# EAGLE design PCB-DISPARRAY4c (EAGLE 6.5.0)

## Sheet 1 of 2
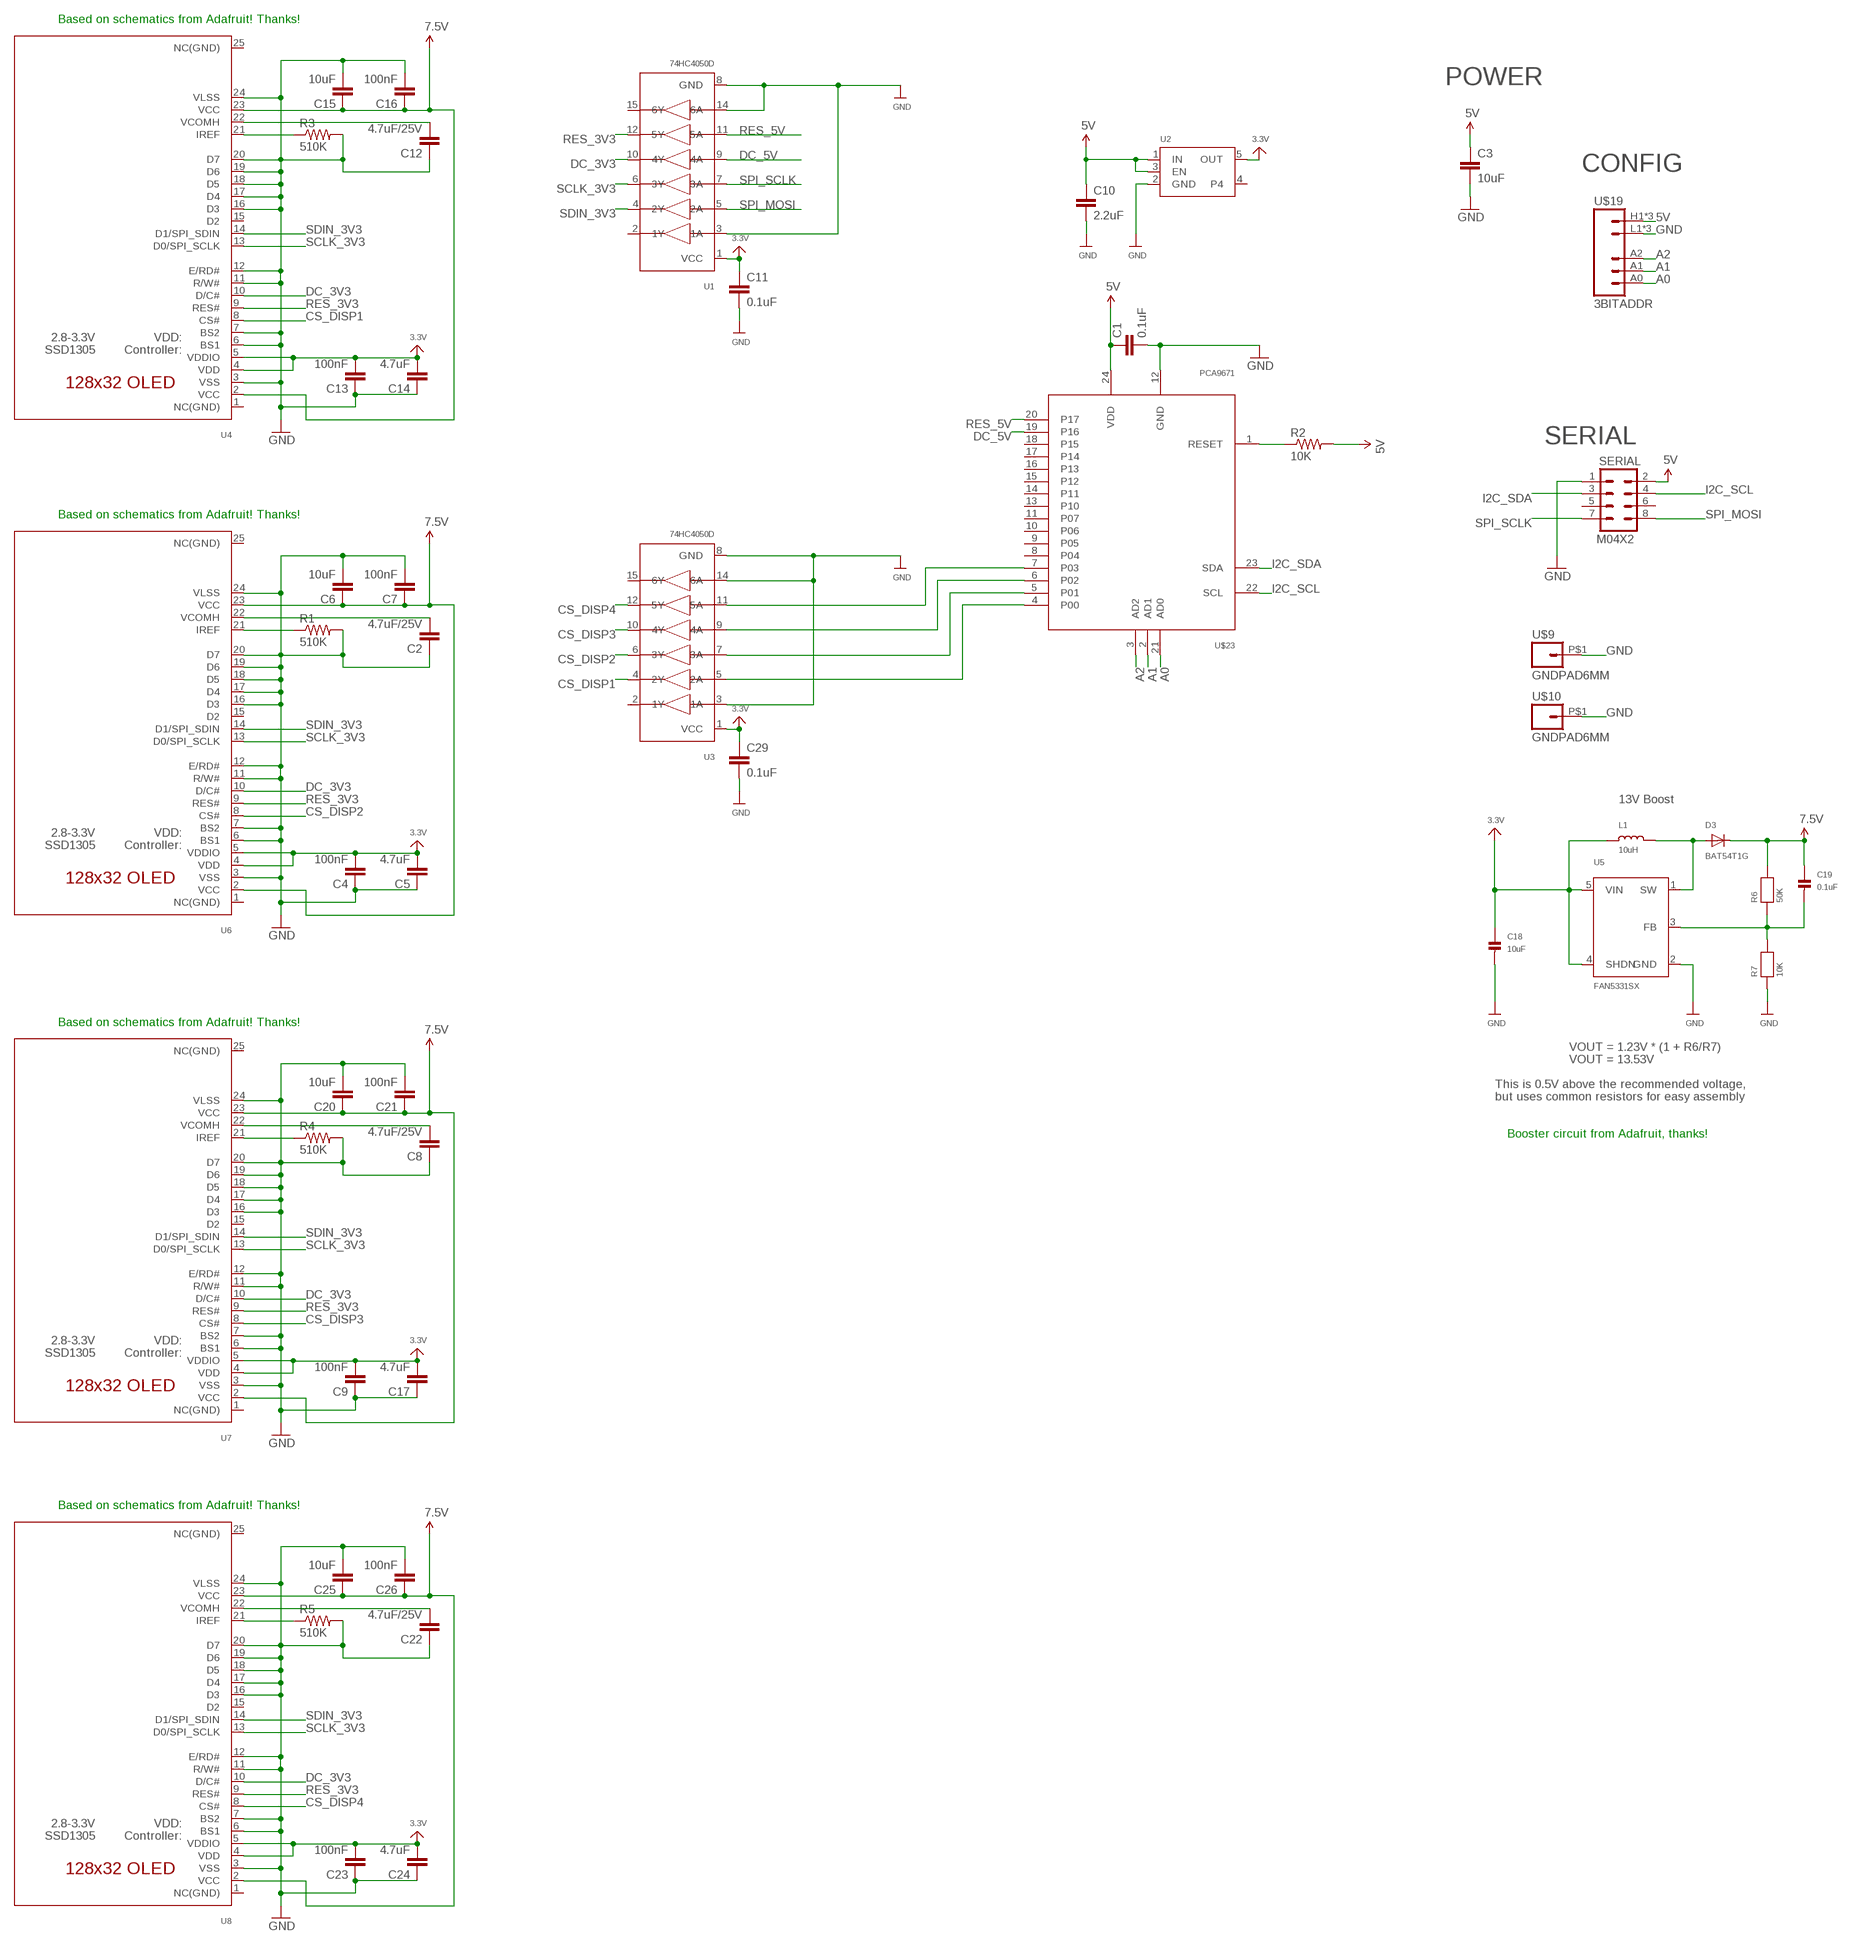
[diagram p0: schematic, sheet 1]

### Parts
C1  0.1uF  CAP0603-CAP  [0603-CAP]
C2  4.7uF/25V  CAP0805  [0805]
C3  10uF  CAP0805  [0805]
C4  100nF  CAP0603-CAP  [0603-CAP]
C5  4.7uF  CAP0603-CAP  [0603-CAP]
C6  10uF  CAP0603-CAP  [0603-CAP]
C7  100nF  CAP0603-CAP  [0603-CAP]
C8  4.7uF/25V  CAP0805  [0805]
C9  100nF  CAP0603-CAP  [0603-CAP]
C10  2.2uF  CAP0603-CAP  [0603-CAP]
C11  0.1uF  CAP0603-CAP  [0603-CAP]
C12  4.7uF/25V  CAP0805  [0805]
C13  100nF  CAP0603-CAP  [0603-CAP]
C14  4.7uF  CAP0603-CAP  [0603-CAP]
C15  10uF  CAP0603-CAP  [0603-CAP]
C16  100nF  CAP0603-CAP  [0603-CAP]
C17  4.7uF  CAP0603-CAP  [0603-CAP]
C18  10uF  CAP_CERAMIC0805  [0805]
C19  0.1uF  CAP_CERAMIC0805  [0805]
C20  10uF  CAP0603-CAP  [0603-CAP]
C21  100nF  CAP0603-CAP  [0603-CAP]
C22  4.7uF/25V  CAP0805  [0805]
C23  100nF  CAP0603-CAP  [0603-CAP]
C24  4.7uF  CAP0603-CAP  [0603-CAP]
C25  10uF  CAP0603-CAP  [0603-CAP]
C26  100nF  CAP0603-CAP  [0603-CAP]
C29  0.1uF  CAP0603-CAP  [0603-CAP]
D3  BAT54T1G  DIODESOD-123  [SOD-123]
L1  10uH  INDUCTOR  [INDUCTOR_1007]
R1  510K  RESISTOR0603-RES  [0603-RES]
R2  10K  RESISTOR0603-RES  [0603-RES]
R3  510K  RESISTOR0603-RES  [0603-RES]
R4  510K  RESISTOR0603-RES  [0603-RES]
R5  510K  RESISTOR0603-RES  [0603-RES]
R6  50K  RESISTOR0805  [0805]
R7  10K  RESISTOR0805  [0805]
SERIAL  M04X2  [2X4]
U1  74HC4050D  74HC4050DTSSOP16  [TSSOP16]
U2  VREG_SOT23-5  [SOT23-5]
U3  74HC4050D  74HC4050DTSSOP16  [TSSOP16]
U4  ER-OLED0.91-2  [ER-OLED0.91-2_WRAPAROUND]
U5  FAN5331SX  FAN5331  [SOT23-5]
U6  ER-OLED0.91-2  [ER-OLED0.91-2_WRAPAROUND]
U7  ER-OLED0.91-2  [ER-OLED0.91-2_WRAPAROUND]
U8  ER-OLED0.91-2  [ER-OLED0.91-2_WRAPAROUND]
U$9  GNDPAD6MM  [3.2MMPAD6MM]
U$10  GNDPAD6MM  [3.2MMPAD6MM]
U$19  3BITADDR  [3BITADDR]
U$23  PCA9671  [TSSOP24]

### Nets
3.3V: C4.2 C5.2 C9.2 C11.1 C13.2 C14.2 C17.2 C18.1 C23.2 C24.2 C29.1 L1.P$1 U1.1(VCC) U2.5(OUT) U3.1(VCC) U4.4(VDD) U4.5(VDDIO) U5.4(SHDN) U5.5(VIN) U6.4(VDD) U6.5(VDDIO) U7.4(VDD) U7.5(VDDIO) U8.4(VDD) U8.5(VDDIO)
5V [Power]: C1.1 C3.1 C10.1 R2.2 SERIAL.2 U2.1(IN) U2.3(EN) U$19.H1(VCC) U$19.H2(VCC) U$19.H3(VCC) U$23.24(VDD)
7.5V [Power]: C6.1 C7.1 C15.1 C16.1 C19.1 C20.1 C21.1 C25.1 C26.1 D3.C R6.2 U4.2(VCC) U4.23(VCC) U6.2(VCC) U6.23(VCC) U7.2(VCC) U7.23(VCC) U8.2(VCC) U8.23(VCC)
A0: U$19.A0 U$23.21(AD0)
A1: U$19.A1 U$23.2(AD1)
A2: U$19.A2 U$23.3(AD2)
CS_DISP1: U3.4(2Y) U4.8(CS#)
CS_DISP2: U3.6(3Y) U6.8(CS#)
CS_DISP3: U3.10(4Y) U7.8(CS#)
CS_DISP4: U3.12(5Y) U8.8(CS#)
DC_3V3: U1.10(4Y) U4.10(D/C#) U6.10(D/C#) U7.10(D/C#) U8.10(D/C#)
DC_5V: U1.9(4A) U$23.19(P16)
GND [Power]: C1.2 C2.1 C3.2 C4.1 C5.1 C6.2 C7.2 C8.1 C9.1 C10.2 C11.2 C12.1 C13.1 C14.1 C15.2 C16.2 C17.1 C18.2 C20.2 C21.2 C22.1 C23.1 C24.1 C25.2 C26.2 C29.2 R1.2 R3.2 R4.2 R5.2 R7.1 SERIAL.1 U1.3(1A) U1.8(GND) U1.14(6A) U2.2(GND) U3.3(1A) U3.8(GND) U3.14(6A) U4.3(VSS) U4.6(BS1) U4.7(BS2) U4.11(R/W#) U4.12(E/RD#) U4.16(D3) U4.17(D4) U4.18(D5) U4.19(D6) U4.20(D7) U4.24(VLSS) U5.2(GND) U6.3(VSS) U6.6(BS1) U6.7(BS2) U6.11(R/W#) U6.12(E/RD#) U6.16(D3) U6.17(D4) U6.18(D5) U6.19(D6) U6.20(D7) U6.24(VLSS) U7.3(VSS) U7.6(BS1) U7.7(BS2) U7.11(R/W#) U7.12(E/RD#) U7.16(D3) U7.17(D4) U7.18(D5) U7.19(D6) U7.20(D7) U7.24(VLSS) U8.3(VSS) U8.6(BS1) U8.7(BS2) U8.11(R/W#) U8.12(E/RD#) U8.16(D3) U8.17(D4) U8.18(D5) U8.19(D6) U8.20(D7) U8.24(VLSS) U$9.P$1 U$10.P$1 U$19.L1(GND) U$19.L2(GND) U$19.L3(GND) U$23.12(GND)
I2C_SCL: SERIAL.4 U$23.22(SCL)
I2C_SDA: SERIAL.3 U$23.23(SDA)
N$1: R2.1 U$23.1(RESET)
N$2: R1.1 U6.21(IREF)
N$3: C2.2 U6.22(VCOMH)
N$4: R4.1 U7.21(IREF)
N$5: R3.1 U4.21(IREF)
N$6: C8.2 U7.22(VCOMH)
N$7: R5.1 U8.21(IREF)
N$8: C22.2 U8.22(VCOMH)
N$10: C12.2 U4.22(VCOMH)
N$14: D3.A L1.P$2 U5.1(SW)
N$15: C19.2 R6.1 R7.2 U5.3(FB)
N$29: U3.5(2A) U$23.4(P00)
N$30: U3.7(3A) U$23.5(P01)
N$31: U3.9(4A) U$23.6(P02)
N$32: U3.11(5A) U$23.7(P03)
RES_3V3: U1.12(5Y) U4.9(RES#) U6.9(RES#) U7.9(RES#) U8.9(RES#)
RES_5V: U1.11(5A) U$23.20(P17)
SCLK_3V3: U1.6(3Y) U4.13(D0/SPI_SCLK) U6.13(D0/SPI_SCLK) U7.13(D0/SPI_SCLK) U8.13(D0/SPI_SCLK)
SDIN_3V3: U1.4(2Y) U4.14(D1/SPI_SDIN) U6.14(D1/SPI_SDIN) U7.14(D1/SPI_SDIN) U8.14(D1/SPI_SDIN)
SPI_MOSI: SERIAL.8 U1.5(2A)
SPI_SCLK: SERIAL.7 U1.7(3A)
Unconnected: SERIAL.5 SERIAL.6 U1.2(1Y) U1.15(6Y) U2.4 U3.2(1Y) U3.15(6Y) U4.1(NC(GND)) U4.15(D2) U4.25(NC(GND)) U6.1(NC(GND)) U6.15(D2) U6.25(NC(GND)) U7.1(NC(GND)) U7.15(D2) U7.25(NC(GND)) U8.1(NC(GND)) U8.15(D2) U8.25(NC(GND)) U$23.8(P04) U$23.9(P05) U$23.10(P06) U$23.11(P07) U$23.13(P10) U$23.14(P11) U$23.15(P12) U$23.16(P13) U$23.17(P14) U$23.18(P15)

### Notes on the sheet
- Based on schematics from Adafruit! Thanks!
- POWER
- CONFIG
- SERIAL
- Based on schematics from Adafruit! Thanks!
- 13V Boost
- Based on schematics from Adafruit! Thanks!
- VOUT = 1.23V * (1 + R6/R7)
- VOUT = 13.53V
- This is 0.5V above the recommended voltage,
- but uses common resistors for easy assembly
- Booster circuit from Adafruit, thanks!
- Based on schematics from Adafruit! Thanks!

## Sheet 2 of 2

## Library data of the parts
C1-C17 C20-C26 C29 = SparkFun:CAP: Capacitor
C18 C19 = microbuilder:CAP_CERAMIC: Ceramic Capacitors
D3 = microbuilder:DIODE: Diode
L1 = microbuilder:INDUCTOR: Inductors
R1-R5 = SparkFun:RESISTOR: Resistor
R6 R7 = microbuilder:RESISTOR: Resistors
SERIAL = SparkFun:M04X2
U1 U3 = SKAARHOJ:74HC4050D: 6-channel level shifter 74HC4050D - 2V-6V Supply Digikey: 74HC4050D,653-ND Mouser: 771-74HC4050D-T
U2 = microbuilder:VREG_SOT23-5: SOT23-5 Fixed Voltage Regulators To better organise some of the SOT23-5 fixed voltage regulators in this library, this new part was created. Part Current Out V Out V In V Dropout Digikey Part No. ADP121 150mA 3.3V 3.4-5.5V 0.09V @ 150mA ADP121-AUJZ33R7CT-ND ADP121 150mA 3.0V 3.1-5.5V 0.09V @ 150mA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
U4 U6-U8 = SKAARHOJ:ER-OLED0.91-2: UG-2864HSWEG01 OLED display Both 1.3" and 0.96" models share the same FPC tab footprint, only the screen dimensions vary.
U5 = microbuilder:FAN5331: FAN5331 - LED/OLED 20V Boost Converter Digikey: FAN5331SXCT-ND
U$9 U$10 = SKAARHOJ:GNDPAD
U$19 = SKAARHOJ:3BITADDR
U$23 = SKAARHOJ:PCA9671

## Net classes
0 default: width 0.203 mm, drill 0.305 mm, clearance 0.152 mm
1 Power: width 0.203 mm, drill 0.406 mm, clearance 0.152 mm

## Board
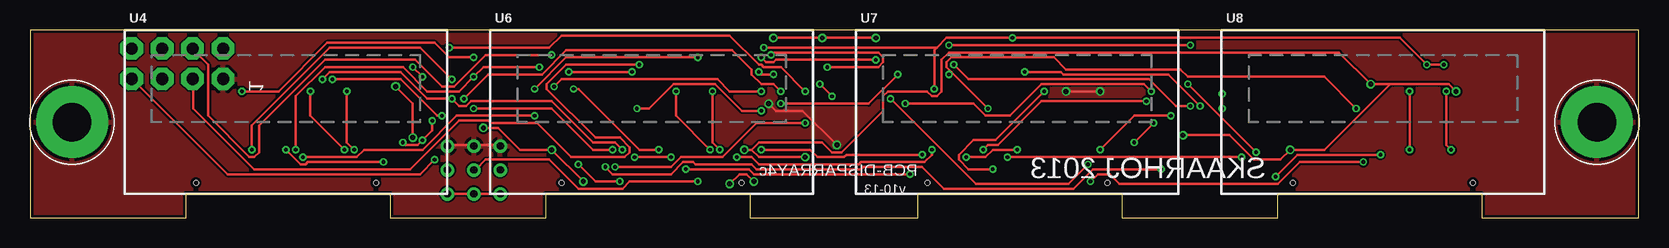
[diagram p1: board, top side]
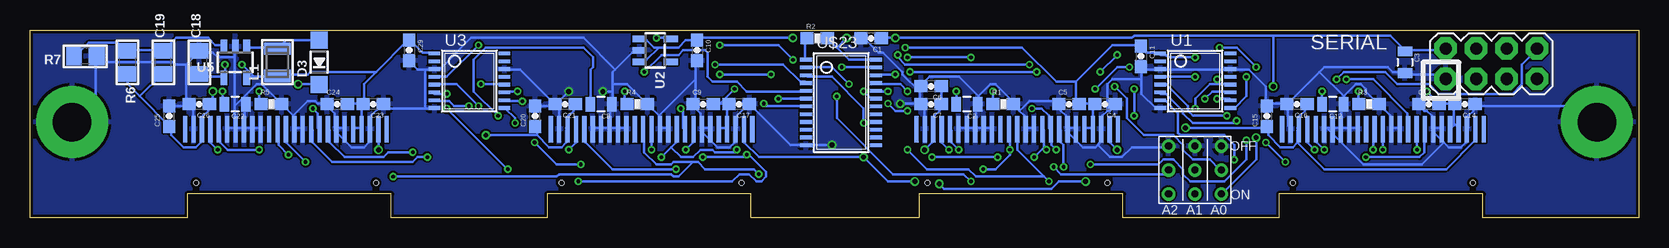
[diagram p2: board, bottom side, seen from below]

Size 134.11 x 15.7 mm. Coordinates in mm from the lower left corner, seen from the top.
Outline: 134.11,0 134.11,15.7 0,15.7 0,0 13,0 13,2 30,2 30,0 43,0 43,2 60,2 60,0 74,0 74,2 91,2 91,0 104,0 104,2 121,2 121,0 134.11,0
Copper layers (1*16): Top 0.035mm / dielectric 1.5mm / Bottom 0.035mm
Design rules "Fusion_eagle_rule_v1.1": minimum track width 6mil, minimum drill 12mil, track to track 6mil, track to pad 6mil, pad to pad 6mil, via to via 6mil, smd to smd 0mil, copper to edge 10mil, drill to drill 10mil, minimum pad ring 10mil, minimum via ring 6mil, stop-mask expansion 2mil, vias tented up to drill 100mil, thermal gap 10mil

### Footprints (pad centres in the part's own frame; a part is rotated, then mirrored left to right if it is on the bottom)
0603-CAP = smd 1.1 x 1: 1 -0.85,0; 2 0.85,0
0805 = smd 0.8 x 1.2: 1 -0.9,0; 2 0.9,0
0805' = smd 1.3 x 1.5: 1 -0.95,0; 2 0.95,0
SOD-123 = smd 1.4 x 1.4: A 1.85,0; C -1.85,0
INDUCTOR_1007 = smd 1.016 x 2.2: P$1 -1.127,0; P$2 1.127,0
0603-RES = smd 1.1 x 1: 1 -0.85,0; 2 0.85,0
2X4 = drill 1.016 pad 1.88 octagon: 1 -3.81,-1.27; 2 -3.81,1.27; 3 -1.27,-1.27; 4 -1.27,1.27; 5 1.27,-1.27; 6 1.27,1.27; 7 3.81,-1.27; 8 3.81,1.27
TSSOP16 = smd 0.305 x 0.991: 1 -3.575,-2.918; 2 -2.925,-2.918; 3 -2.275,-2.918; 4 -1.625,-2.918; 5 -0.975,-2.918; 6 -0.325,-2.918; 7 0.325,-2.918; 8 0.975,-2.918; 9 0.975,2.918; 10 0.325,2.918; 11 -0.325,2.918; 12 -0.975,2.918; 13 -1.625,2.918; 14 -2.275,2.918; 15 -2.925,2.918; 16 -3.575,2.918
SOT23-5 = smd 0.55 x 1.2: 1 -0.95,-1.3; 2 0,-1.3; 3 0.95,-1.3; 4 0.95,1.3; 5 -0.95,1.3
ER-OLED0.91-2_WRAPAROUND = smd 0.35 x 2.2 bottom: 1 -8.4,-1.43; 2 -7.7,-1.43; 3 -7,-1.43; 4 -6.3,-1.43; 5 -5.6,-1.43; 6 -4.9,-1.43; 7 -4.2,-1.43; 8 -3.5,-1.43; 9 -2.8,-1.43; 10 -2.1,-1.43; 11 -1.4,-1.43; 12 -0.7,-1.43; 13 0,-1.43; 14 0.7,-1.43; 15 1.4,-1.43; 16 2.1,-1.43; 17 2.8,-1.43; 18 3.5,-1.43; 19 4.2,-1.43; 20 4.9,-1.43; 21 5.6,-1.43; 22 6.3,-1.43; 23 7,-1.43; 24 7.7,-1.43; 25 8.4,-1.43 | hole 0.4: -7.5,-5.93; 7.5,-5.93
3.2MMPAD6MM = drill 3.2 pad 6: P$1 0,0
3BITADDR = drill 0.6: A0 -2.2,0; A1 0,0; A2 2.2,0; H1 -2.2,2; H2 0,2; H3 2.2,2; L1 -2.2,-2; L2 0,-2; L3 2.2,-2
TSSOP24 = smd 0.305 x 0.991: 1 -4.225,-2.918; 2 -3.575,-2.918; 3 -2.925,-2.918; 4 -2.275,-2.918; 5 -1.625,-2.918; 6 -0.975,-2.918; 7 -0.325,-2.918; 8 0.325,-2.918; 9 0.975,-2.918; 10 1.625,-2.918; 11 2.275,-2.918; 12 2.925,-2.918; 13 2.925,2.918; 14 2.275,2.918; 15 1.625,2.918; 16 0.975,2.918; 17 0.325,2.918; 18 -0.325,2.918; 19 -0.975,2.918; 20 -1.625,2.918; 21 -2.275,2.918; 22 -2.925,2.918; 23 -3.575,2.918; 24 -4.225,2.918

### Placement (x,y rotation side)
C1  64,15 180 bottom
C2  56,9.5 180 bottom
C3  19.5,13 270 bottom
C4  44.5,9.5 180 bottom
C5  47.5,9.5 0 bottom
C6  59,11 180 bottom
C7  59,9.5 180 bottom
C8  86.5,9.5 180 bottom
C9  78,9.5 0 bottom
C10  78.5,14 270 bottom
C11  41.5,13.5 270 bottom
C12  25.5,9.5 180 bottom
C13  17.5,9.5 0 bottom
C14  14.5,9.5 180 bottom
C15  31,8.5 90 bottom
C16  28.5,9.5 180 bottom
C17  75,9.5 180 bottom
C18  10uF  [0805']  120,13 90 bottom
C19  0.1uF  [0805']  123,13 90 bottom
C20  92,8.5 90 bottom
C21  89.5,9.5 180 bottom
C22  117,9.5 180 bottom
C23  105.5,9.5 180 bottom
C24  108.5,9.5 0 bottom
C25  122.5,8.5 90 bottom
C26  120,9.5 180 bottom
C29  102.5,14 270 bottom
D3  110,13 90 bottom
L1  113.5,13 90 bottom
R1  53,9.5 0 bottom
R2  68.5,15 0 bottom
R3  22.5,9.5 0 bottom
R4  83.5,9.5 0 bottom
R5  114,9.5 0 bottom
R6  50K  [0805']  126,13 270 bottom
R7  10K  [0805']  129.5,13.5 180 bottom
SERIAL  12.29,12.88 0 bottom
U1  36.98,10.16 270 bottom
U2  82,14 270 bottom
U3  97.49,10.16 270 bottom
U4  21.34,8.85 0 top
U5  117,13 180 bottom
U6  51.82,8.85 0 top
U7  82.3,8.85 0 top
U8  112.78,8.85 0 top
U$9  130.61,8 0 top
U$10  3.5,8 0 top
U$19  37,4 180 bottom
U$23  66.5,8.99 270 bottom

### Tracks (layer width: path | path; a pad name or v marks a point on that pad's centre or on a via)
3.3V  (via drill 0.3)
  Top 0.203: v17.68,10.57 20.73,10.57 24.79,14.63 33.73,14.63 34.95,13.41 v36.98,13.41 | 75.59,14.22 75.39,14.02 v75.39,10.77 | 75.59,14.22 76.4,15.04 v81.89,15.04 114.2,15.04 v116.43,12.8 v117.86,12.8 | 75.59,14.22 v61.16,14.22
  Bottom 0.203: 15.44,7.92 15.44,7.72 15.65,7.52 U4.5 | 15.44,7.92 15.44,9.35 C14.2 15.44,9.55 16.46,9.55 C13.2 16.66,9.55 v17.68,10.57 | 15.44,7.92 15.04,7.52 U4.4 | 45.52,7.52 45.52,9.35 C4.2 45.52,9.55 46.53,9.55 C5.2 46.74,9.55 46.94,9.75 46.94,11.38 | 46.94,11.38 43.89,14.43 41.66,14.43 C11.1 41.45,14.22 41.05,13.82 40.03,13.82 U1.1 39.83,13.61 39.42,13.61 39.22,13.41 v36.98,13.41 | 45.52,7.52 46.13,7.52 U6.5 | 45.52,7.52 U6.4 | 76,7.52 76.61,7.52 U7.5 | 76.61,9.55 77.01,9.55 C9.2 76.61,9.55 | 76.61,9.55 76,9.55 C17.2 76,9.35 76,7.52 | v81.89,15.04 80.87,15.04 U2.5 | 76.61,9.55 v75.39,10.77 | 76,7.52 U7.4 | C18.1 119.89,11.99 119.69,11.79 118.06,11.79 U5.4 117.86,11.79 v117.86,12.8 | 115.42,11.79 113.59,11.79 L1.P$1 113.39,11.99 110.95,11.99 110.74,12.19 105.26,12.19 | 115.42,11.79 116.03,11.79 U5.5 | 115.42,11.79 v116.43,12.8 | U3.1 100.58,13.82 101.4,13.82 102.41,14.83 C29.1 102.62,14.83 105.26,12.19 | C23.2 106.48,9.55 107.49,9.55 C24.2 | 106.48,7.52 106.48,9.35 C23.2 | 105.26,12.19 106.27,11.18 106.27,9.55 C23.2 | 106.48,7.52 107.09,7.52 U8.5 | 106.48,7.52 U8.4 | 46.94,11.38 48.56,11.38 51.41,14.22 v61.16,14.22
5V  (via drill 0.41)
  Top 0.203: U$19.H1 34.95,2.03 36.98,2.03 U$19.H2 37.19,2.03 39.01,2.03 U$19.H3 | v61.98,15.04 v66.04,15.04 v70.51,15.04 | v31.9,6.71 31.9,9.55 v30.48,10.97
  Bottom 0.203: 81.69,14.22 82.09,14.22 82.7,14.83 83.11,14.83 U2.1 | 81.69,14.22 80.06,14.22 79.45,14.83 78.64,14.83 C10.1 78.44,15.04 v70.51,15.04 | 81.69,14.22 82.7,13.21 83.11,13.21 U2.3 | 66.85,14.22 67.46,14.83 R2.2 | 66.85,14.22 65.84,13.21 63.6,13.21 U$23.24 | 30.48,15.24 20.73,15.24 19.51,14.02 C3.1 19.3,14.02 16.26,14.02 SERIAL.2 | 30.48,15.24 42.06,15.24 42.27,15.04 v61.98,15.04 62.99,15.04 C1.1 | v66.04,15.04 66.85,14.22 | v31.9,6.71 31.9,4.88 34.75,2.03 U$19.H1 | 30.48,15.24 v30.48,10.97
7.5V  (via drill 0.41)
  Top 0.203: v37.8,7.52 39.01,7.52 40.84,5.69 v43.48,5.69 v46.13,3.05 | v64.62,5.08 60.76,5.08 60.15,5.69 | v59.54,5.69 60.15,5.69 | 113.39,11.18 118.26,11.18 v118.87,10.57 | 113.39,11.18 v111.76,11.18 109.12,13.82 76.61,13.82 76,13.21 76,10.57 75.59,10.16 75.18,10.16 74.78,10.57 71.53,10.57 71.12,10.16 71.12,8.94 67.67,5.49 66.85,5.49 66.04,6.3 60.76,6.3 60.15,5.69 | 113.39,11.18 107.9,5.69 v105.05,5.69 104.24,4.88 102.01,4.88 99.97,6.91 v96.11,6.91 | v58.32,2.85 59.13,3.66 59.74,3.66 v60.35,3.05
  Bottom 0.203: 44.09,7.52 U6.2 44.09,7.32 44.09,6.3 v43.48,5.69 | 28.45,6.3 28.85,5.89 29.87,5.89 30.89,6.91 30.89,7.52 C15.1 31.09,7.52 v37.8,7.52 | 28.45,6.3 28.45,7.32 U4.23 | C16.1 27.84,9.35 27.84,8.94 28.25,8.53 28.25,7.52 U4.23 | 28.45,6.3 26.21,4.06 16.05,4.06 13.61,6.5 13.61,7.32 U4.2 | 28.45,7.52 U4.23 | 74.57,7.52 U7.2 74.57,7.32 74.57,6.3 73.36,5.08 v64.62,5.08 62.59,3.05 v60.35,3.05 | C6.1 58.12,10.97 58.12,9.55 C7.1 58.32,9.35 58.32,8.94 58.73,8.53 58.73,7.52 U6.23 | 58.93,7.52 U6.23 | v59.54,5.69 58.93,6.3 58.93,7.32 U6.23 | 124.97,10.16 125.98,11.18 125.98,11.99 R6.2 | 124.97,10.16 122.53,7.72 C25.1 122.33,7.52 122.33,6.91 121.31,5.89 120.29,5.89 119.89,6.3 119.89,7.32 U8.23 | 124.97,10.16 123.14,11.99 C19.1 | 91.85,6.91 91.85,7.52 C20.1 | 91.85,6.91 90.83,5.89 89.81,5.89 89.41,6.3 89.41,7.32 U7.23 | C21.1 88.8,9.35 88.8,8.94 89.2,8.53 89.2,7.52 U7.23 | 89.41,7.52 U7.23 | 105.05,7.52 U8.2 105.05,7.32 v105.05,5.69 | U8.23 119.69,7.52 119.69,8.53 119.28,8.94 119.28,9.35 C26.1 119.08,9.55 118.87,9.75 v118.87,10.57 | v111.76,11.18 110.13,11.18 D3.C | 119.89,7.52 U8.23 | v96.11,6.91 91.85,6.91 | v46.13,3.05 48.36,3.05 48.97,2.44 57.91,2.44 v58.32,2.85
A0  (via drill 0.3)
  Top 0.203: v60.96,10.57 58.32,10.57 57.3,11.58 44.3,11.58 v43.69,10.97
  Bottom 0.203: v60.96,10.57 61.57,11.18 63.4,11.18 U$23.21 | v43.69,10.97 42.67,9.96 42.67,8.33 41.25,6.91 38.81,6.91 38,6.1 38,5.69 37.19,4.88 35.76,4.88 34.95,4.06 U$19.A0
A1  (via drill 0.3)
  Top 0.203: v66.85,10.16 v65.84,11.18 | v55.68,3.05 49.99,3.05 49.38,2.44 45.72,2.44 43.28,4.88 38,4.88 37.19,4.06 U$19.A1
  Bottom 0.203: v65.84,11.18 67.26,12.6 69.29,12.6 U$23.2 | v66.85,10.16 66.85,8.33 62.18,3.66 56.29,3.66 v55.68,3.05
A2  (via drill 0.3)
  Top 0.203: v64.62,7.92 60.55,7.92 57.71,5.08 54.25,5.08 53.44,4.27 v48.77,4.27
  Bottom 0.203: v64.62,7.92 64.62,9.14 67.26,11.79 69.29,11.79 U$23.3 | v48.77,4.27 48.16,3.66 39.42,3.66 39.22,3.86 U$19.A2
CS_DISP1  (via drill 0.3)
  Top 0.203: v76.61,14.43 v96.72,14.43 | v70.51,13.21 62.18,13.21 61.98,13.01 61.37,13.01 v60.96,13.41 | v55.68,13.41 44.7,13.41 v42.06,10.77 | v42.06,8.53 35.56,8.53 32.72,5.69 27.84,5.69 27.23,5.08 v22.76,5.08
  Bottom 0.203: v96.72,14.43 99.36,11.79 100.38,11.79 U3.4 | v76.61,14.43 71.73,14.43 v70.51,13.21 | v55.68,13.41 v60.96,13.41 | v42.06,8.53 v42.06,10.77 | v22.76,5.08 18.29,5.08 17.88,5.49 17.88,7.32 U4.8
CS_DISP2  (via drill 0.3)
  Top 0.203: v99.36,9.14 v99.36,10.36 | v94.28,4.06 88.59,4.06 86.97,2.44 76.2,2.44 74.37,4.27 69.49,4.27 69.29,4.06 60.55,4.06 60.15,4.47 55.47,4.47 55.27,4.67 54.46,4.67 53.44,3.66 48.56,3.66 v47.95,4.27
  Bottom 0.203: v99.36,10.36 100.38,10.36 U3.6 | v94.28,4.06 v99.36,9.14 | v47.95,4.27 47.95,6.1 48.16,6.3 48.16,7.32 U6.8
CS_DISP3  (via drill 0.3)
  Top 0.203: v93.07,9.75 84.33,9.75 80.67,6.1 79.86,6.1 v79.45,5.69
  Bottom 0.203: v93.07,9.75 94.49,9.75 U3.10 | v79.45,5.69 78.84,6.3 78.84,7.32 U7.8
CS_DISP4  (via drill 0.3)
  Top 0.203: v102.21,5.49 v96.52,11.18
  Bottom 0.203: v96.52,11.18 94.69,11.18 U3.12 | v102.21,5.49 104.24,5.49 104.65,5.08 107.9,5.08 109.12,6.3 109.12,7.32 U8.8
DC_3V3  (via drill 0.3)
  Top 0.203: v100.99,5.08 v81.48,5.08 | v24.38,11.58 24.99,12.19 30.89,12.19 33.12,9.96 v35.15,9.96 35.76,9.35 36.37,9.35 36.78,9.75 43.48,9.75 46.94,6.3 48.77,6.3 v49.38,5.69 | v75.18,5.69 75.18,5.28 74.57,4.67 69.29,4.67 69.09,4.47 60.76,4.47 60.15,5.08 v58.93,5.08 | v50.39,5.08 v53.44,5.08
  Bottom 0.203: v81.48,5.08 80.67,5.89 | 80.67,5.89 80.26,6.3 80.26,7.32 U7.10 | v100.99,5.08 101.8,5.08 102.21,4.67 108.92,4.67 110.54,6.3 110.54,7.32 U8.10 | v35.15,9.96 34.14,9.96 U1.10 | v24.38,11.58 22.15,11.58 19.3,8.74 19.3,7.52 U4.10 | 49.58,5.89 49.58,7.32 U6.10 | 80.67,5.89 79.86,5.08 78.84,5.08 78.23,5.69 77.22,5.69 77.01,5.49 75.39,5.49 v75.18,5.69 | v53.44,5.08 v58.93,5.08 | 49.58,5.89 v50.39,5.08 | 49.58,5.89 v49.38,5.69
DC_5V  (via drill 0.3)
  Top 0.203: v31.9,12.6 v32.72,11.79 | v34.95,14.22 43.28,14.22 44.3,15.24 58.32,15.24 60.76,12.8 60.96,12.8 61.16,12.6 62.59,12.6 v64.62,10.57
  Bottom 0.203: v32.72,11.79 32.72,10.16 33.73,9.14 33.93,9.14 U1.9 | v31.9,12.6 33.53,14.22 v34.95,14.22 | v64.62,10.57 64.01,9.96 63.6,9.96 U$23.19
GND  (via drill 0.41)
  Top 0.203: v86.36,10.57 v89.2,10.57 | U$19.L1 34.95,6.1 36.98,6.1 U$19.L2 37.19,6.1 39.01,6.1 U$19.L3 | v67.26,6.1 64.41,8.94 62.18,8.94 v61.57,9.55
  Bottom 0.203: U3.14 94.49,12.39 93.27,12.39 90.42,9.55 C21.2 | C20.2 91.85,9.35 90.42,9.35 C21.2 | U7.24 90.02,7.52 90.02,9.14 90.22,9.35 C21.2 | U7.16 84.53,7.52 84.94,7.52 U7.17 85.14,7.52 85.75,7.52 | 85.75,7.52 85.75,9.35 C8.1 85.55,9.55 85.55,10.57 | 85.34,12.39 85.55,12.19 85.55,11.18 | 85.34,12.39 83.92,13.82 83.31,13.82 U2.2 | 85.55,10.57 85.55,11.18 | U7.20 87.17,7.52 86.56,7.52 U7.19 86.36,7.52 85.95,7.52 U7.18 85.75,7.52 | v89.2,10.57 90.22,9.55 C21.2 | 85.55,10.57 v86.36,10.57 | 81.69,8.53 82.5,9.35 R4.2 82.7,9.55 84.33,11.18 85.55,11.18 | 81.69,8.53 81.69,7.52 U7.12 81.48,7.52 80.87,7.52 U7.11 | 78.64,9.14 78.23,8.74 78.23,7.52 U7.7 | 78.64,9.14 78.84,9.35 C9.1 78.64,9.14 | 78.64,9.14 78.64,11.58 | 78.64,11.58 78.64,13.01 C10.2 | U7.6 77.42,7.52 78.03,7.52 U7.7 | 78.64,11.58 81.69,8.53 | U7.7 78.23,7.32 76.81,5.89 75.79,5.89 75.39,6.3 75.39,7.32 U7.3 75.18,7.52 75.18,8.53 74.17,9.55 C17.1 73.97,9.35 70.71,6.1 69.49,6.1 U$23.12 69.29,6.1 v67.26,6.1 | 101.19,12.39 101.8,12.39 102.41,13.01 C29.2 | 101.19,12.39 100.58,12.39 U3.3 100.38,12.39 99.97,12.39 97.33,15.04 87.99,15.04 85.34,12.39 | 101.19,9.14 104.44,9.14 104.65,9.35 C23.1 104.85,9.35 105.66,8.53 105.66,7.52 U8.3 105.87,7.32 105.87,6.3 106.27,5.89 107.29,5.89 108.71,7.32 U8.7 | 101.19,9.14 100.58,9.14 U3.8 | 101.19,9.14 101.19,12.39 | 121.11,9.35 120.9,9.35 C26.2 | 121.11,9.35 122.33,9.35 C25.2 | 121.11,12.8 120.09,13.82 C18.2 119.89,13.82 118.87,13.82 118.47,13.41 117.04,13.41 | 121.11,9.35 121.11,12.8 | 121.11,9.35 C26.2 | U8.24 120.5,7.52 120.5,9.14 120.7,9.35 C26.2 | U8.7 108.71,7.52 108.71,8.74 109.32,9.35 C24.1 109.53,9.55 110.13,9.55 110.34,9.75 110.95,9.75 112.17,8.53
  Bottom 0.203: U8.6 107.9,7.52 108.51,7.52 U8.7 | 112.17,8.53 112.98,9.35 R5.2 113.18,9.55 114.81,11.18 115.21,11.18 117.04,9.35 | 112.17,8.53 112.17,7.52 U8.12 111.96,7.52 111.35,7.52 U8.11 | U8.16 115.01,7.52 115.42,7.52 U8.17 115.62,7.52 116.23,7.52 | 116.23,7.52 116.23,9.35 C22.1 | 116.23,7.52 U8.18 116.43,7.52 116.84,7.52 U8.19 117.04,7.52 | 117.04,7.52 117.04,9.35 | 117.04,9.35 117.04,13.41 | 117.04,13.41 117.04,14.22 U5.2 | 117.04,7.52 117.65,7.52 U8.20 | 128.63,13.01 128.63,9.96 130.45,8.13 U$9.P$1 | 128.63,13.01 128.63,13.41 R7.1 128.63,13.01 | 121.11,12.8 121.92,12.8 122.12,13.01 128.63,13.01 | C13.1 18.29,9.35 17.88,8.94 17.68,8.94 17.27,8.53 17.27,7.52 U4.7 | U4.6 16.46,7.52 17.07,7.52 U4.7 | 16.26,6.3 17.27,7.32 U4.7 | 16.26,6.3 15.85,5.89 14.83,5.89 14.43,6.3 14.43,7.32 U4.3 14.22,7.52 14.22,8.53 13.82,8.94 13.82,9.35 C14.1 13.61,9.35 4.88,9.35 3.66,8.13 U$10.P$1 | U4.11 19.91,7.52 20.52,7.52 U4.12 20.73,7.52 20.73,8.53 21.54,9.35 R3.2 21.74,9.55 22.76,10.57 22.76,10.77 23.16,11.18 23.57,11.18 24.59,10.16 | U4.16 23.57,7.52 23.98,7.52 U4.17 24.18,7.52 24.79,7.52 | 24.79,7.52 24.79,9.35 C12.1 24.59,9.55 24.59,10.16 | 26.01,7.52 25.6,7.52 U4.19 25.4,7.52 24.99,7.52 U4.18 24.79,7.52 | 26.01,7.52 26.21,7.52 U4.20 | SERIAL.1 16.26,11.79 16.46,11.99 19.3,11.99 C3.2 19.51,12.19 20.52,12.19 20.93,12.6 26.21,12.6 26.62,12.19 | C16.2 29.46,9.55 30.89,9.55 C15.2 31.09,9.55 31.09,10.97 32.51,12.39 33.93,12.39 U1.14 34.14,12.39 39.83,12.39 U1.3 40.03,12.39 41.45,12.39 | C16.2 29.26,9.35 29.26,7.72 29.06,7.52 U4.24 | 41.45,12.39 41.45,12.6 C11.2 41.45,12.39 | 41.45,12.39 41.45,11.58
  Bottom 0.203: 41.45,11.58 41.45,10.36 40.23,9.14 40.03,9.14 U1.8 | 26.62,12.19 29.26,9.55 C16.2 | 26.62,12.19 24.59,10.16 | 59.94,10.57 59.94,10.97 C6.2 | 59.94,10.57 59.94,9.55 | 59.94,10.57 61.37,11.99 61.37,12.19 62.99,13.82 63.4,13.82 64.41,14.83 64.82,14.83 C1.2 | 59.94,10.57 C6.2 | U6.24 59.54,7.52 59.54,9.14 59.74,9.35 C7.2 59.94,9.55 | U6.16 54.05,7.52 54.46,7.52 U6.17 54.66,7.52 55.27,7.52 | 55.27,7.52 55.27,9.35 C2.1 55.07,9.55 55.07,10.16 | U6.20 56.69,7.52 56.08,7.52 U6.19 55.88,7.52 55.47,7.52 U6.18 55.27,7.52 | 51.61,8.94 51.21,8.53 51.21,7.52 U6.12 51,7.52 50.39,7.52 U6.11 | 51.61,8.94 52.02,9.35 R1.2 52.02,9.55 53.65,11.18 54.05,11.18 55.07,10.16 | 44.3,8.94 44.09,8.94 43.69,9.35 C4.1 | 44.3,8.94 44.7,8.53 44.7,7.52 U6.3 44.91,7.32 44.91,6.3 45.11,6.1 | U6.7 47.75,7.52 47.75,8.53 48.16,8.94 48.16,9.35 C5.1 48.36,9.55 48.56,9.75 50.8,9.75 51.61,8.94 | U6.6 46.94,7.52 47.55,7.52 U6.7 | 45.11,6.1 45.31,5.89 46.33,5.89 47.75,7.32 U6.7 | 45.11,6.1 44.09,5.08 43.08,5.08 42.27,5.89 39.22,5.89 U$19.L3 | 55.07,10.16 56.69,11.79 59.13,11.79 59.74,11.18 C6.2 | 41.45,11.58 43.89,11.58 44.3,11.18 44.3,8.94 | 16.26,6.3 18.09,4.47 22.96,4.47 26.01,7.52 | 59.94,9.55 v61.57,9.55
  pour Top: 0,0 134,0 134,16 0,16
  pour Bottom: 0,0 134,0 134,16 0,16
I2C_SCL  (via drill 0.3)
  Top 0.203: v61.98,11.99 60.96,11.99 v60.76,12.19 | v44.91,12.19 v50.19,12.19 | v43.48,13.61 38,13.61 35.36,10.97 34.34,10.97 32.11,13.21 24.59,13.21 19.1,7.72 19.1,5.49 18.69,5.08 18.29,5.08 14.83,8.53 14.83,12.8 13.61,14.02 SERIAL.4
  Bottom 0.203: v61.98,11.99 63.4,11.99 U$23.22 | v50.19,12.19 v60.76,12.19 | v43.48,13.61 v44.91,12.19
I2C_SDA  (via drill 0.3)
  Top 0.203: v66.45,12.6 70.71,12.6 71.12,13.01 71.12,13.41 70.71,13.82 61.98,13.82 v61.77,13.61 | v50.8,12.8 44.7,12.8 43.08,11.18 43.08,10.77 47.14,6.71 49.17,6.71 49.99,5.89 49.99,5.49 49.58,5.08 45.11,5.08 42.27,7.92 38.41,7.92 38.2,8.13 35.76,8.13 31.7,4.06 18.69,4.06 13.61,9.14 13.61,11.58 SERIAL.3
  Bottom 0.203: v66.45,12.6 63.6,12.6 U$23.23 | v61.77,13.61 61.77,13.41 61.16,12.8 v50.8,12.8
N$1
  Bottom 0.203: U$23.1 69.49,13.21 69.49,14.83 R2.1
N$2  (via drill 0.3)
  Top 0.203: v53.85,10.57 53.85,8.53 v56.69,5.69
  Bottom 0.203: v53.85,10.57 53.85,9.55 R1.1 | v56.69,5.69 57.3,6.3 57.3,7.32 U6.21
N$3  (via drill 0.3)
  Top 0.203: v56.9,10.57 56.9,6.3 v57.51,5.69
  Bottom 0.203: v56.9,10.57 56.9,9.55 C2.2 | v57.51,5.69 58.12,6.3 58.12,7.32 U6.22
N$4  (via drill 0.3)
  Top 0.203: v84.53,10.57 80.47,6.5 78.64,6.5 77.42,5.28 77.42,4.88 78.23,4.06 v80.26,4.06
  Bottom 0.203: v84.53,10.57 84.53,9.55 R4.1 | v80.26,4.06 85.55,4.06 87.78,6.3 87.78,7.32 U7.21
N$5  (via drill 0.3)
  Top 0.203: v23.37,10.57 23.37,8.53 v26.21,5.69
  Bottom 0.203: v23.37,10.57 23.37,9.55 R3.1 | v26.21,5.69 26.82,6.3 26.82,7.32 U4.21
N$6  (via drill 0.3)
  Top 0.203: v95.1,8.53 92.05,8.53 v89.2,5.69
  Bottom 0.203: v95.1,8.53 97.13,10.57 97.13,13.21 96.11,14.22 87.99,14.22 87.17,13.41 87.17,12.6 87.38,12.39 87.38,9.55 C8.2 | v89.2,5.69 88.59,6.3 88.59,7.32 U7.22
N$7  (via drill 0.3)
  Top 0.203: v115.01,5.69 v115.01,10.57
  Bottom 0.203: v115.01,10.57 115.01,9.55 R5.1 | v115.01,5.69 117.65,5.69 118.26,6.3 118.26,7.32 U8.21
N$8  (via drill 0.3)
  Top 0.203: v118.06,10.57 118.06,6.1 v118.47,5.69
  Bottom 0.203: v118.06,10.57 118.06,9.55 C22.2 | v118.47,5.69 119.08,6.3 119.08,7.32 U8.22
N$10  (via drill 0.3)
  Top 0.203: v26.42,10.57 26.42,6.3 v27.03,5.69
  Bottom 0.203: v26.42,10.57 26.42,9.55 C12.2 | v27.03,5.69 27.64,6.3 27.64,7.32 U4.22
N$14
  Bottom 0.203: U5.1 116.03,14.22 113.59,14.22 L1.P$2 113.39,14.22 112.78,14.83 110.13,14.83 D3.A
N$15
  Bottom 0.203: U5.3 118.06,14.43 118.67,14.43 119.28,15.04 121.92,15.04 122.94,14.02 C19.2 123.14,14.02 125.98,14.02 R6.1 126.19,14.02 126.8,14.63 129.24,14.63 130.25,13.61 R7.2
N$29  (via drill 0.3)
  Top 0.203: v96.72,9.35 95.5,9.35 93.27,11.58 78.23,11.58 v77.01,12.8
  Bottom 0.203: v96.72,9.35 98.55,11.18 100.38,11.18 U3.5 | v77.01,12.8 71.32,12.8 69.9,11.38 69.49,11.38 U$23.4
N$30  (via drill 0.3)
  Top 0.203: v82.91,12.19 85.95,12.19 86.16,11.99 94.89,11.99 v97.54,9.35
  Bottom 0.203: v82.91,12.19 81.48,13.61 80.06,13.61 79.65,14.02 77.83,14.02 77.62,13.82 77.62,11.79 77.22,11.38 75.18,11.38 74.37,10.57 69.49,10.57 U$23.5 | v97.54,9.35 98.75,9.35 99.16,9.75 100.38,9.75 U3.7
N$31  (via drill 0.3)
  Top 0.203: v71.73,9.96 78.84,2.85 86.56,2.85 v88.19,4.47 | v93.67,7.92 v92.05,6.3
  Bottom 0.203: v71.73,9.96 69.49,9.96 U$23.6 | v88.19,4.47 90.22,4.47 v92.05,6.3 | v93.67,7.92 93.67,8.33 94.49,9.14 U3.9
N$32  (via drill 0.3)
  Top 0.203: v72.95,9.55 78.64,9.55 79.65,8.53 81.69,8.53 84.33,11.18 92.86,11.18 v93.47,10.57
  Bottom 0.203: v72.95,9.55 72.75,9.35 69.49,9.35 U$23.7 | v93.47,10.57 94.49,10.57 U3.11
RES_3V3  (via drill 0.3)
  Top 0.203: v36.98,9.14 43.48,9.14 46.94,5.69 v48.56,5.69 | v18.49,5.69 18.49,7.72 24.99,14.22 32.51,14.22 v35.15,11.58 | 76.81,12.19 76.4,12.6 76.4,13.01 76.81,13.41 85.34,13.41 86.36,12.39 95.91,12.39 96.52,11.79 107.9,11.79 v110.54,9.14 | 76.81,12.19 v79.86,9.14 | v50.6,9.14 51.61,9.14 53.65,11.18 57.1,11.18 59.33,8.94 v60.96,8.94 | v62.59,9.55 69.9,9.55 v72.34,11.99 | 76.81,12.19 v76.61,11.99
  Bottom 0.203: 35.15,11.18 35.76,11.18 36.98,9.96 v36.98,9.14 | 35.15,11.18 34.14,11.18 U1.12 | v48.56,5.69 48.97,6.1 48.97,7.32 U6.9 49.17,7.52 49.17,8.53 49.78,9.14 v50.6,9.14 | v18.49,5.69 18.49,7.32 U4.9 | 35.15,11.18 v35.15,11.58 | v79.86,9.14 79.65,8.94 79.65,7.52 U7.9 | v110.54,9.14 110.13,8.74 110.13,7.52 U8.9 | v60.96,8.94 61.98,8.94 v62.59,9.55 | v76.61,11.99 v72.34,11.99
RES_5V  (via drill 0.3)
  Top 0.203: v36.17,9.96 38.2,11.99 42.67,11.99 44.7,14.02 58.52,14.02 60.15,12.39 60.15,11.99 60.96,11.18 61.98,11.18 v62.59,10.57
  Bottom 0.203: v36.17,9.96 35.56,10.57 34.14,10.57 U1.11 | v62.59,10.57 63.4,10.57 U$23.20
SCLK_3V3  (via drill 0.3)
  Top 0.203: v33.53,8.13 33.53,7.32 v32.72,6.5 32.31,6.1 31.29,6.1 v31.09,6.3 | v29.46,4.67 23.16,4.67 22.96,4.47 22.55,4.47 v21.34,5.69 | v49.17,3.05 47.14,3.05 v45.72,4.47 | v82.3,5.69 80.26,5.69 79.65,5.08 v78.03,5.08 | v74.37,5.28 68.07,5.28 67.87,5.08 65.63,5.08 65.02,5.69 v60.96,5.69 | v111.15,4.67 105.87,4.67 104.04,2.85 90.83,2.85 90.02,3.66 89,3.66 v88.39,3.05
  Bottom 0.203: v33.53,8.13 33.73,7.92 37.19,7.92 38,8.74 38,8.94 39.42,10.36 39.83,10.36 U1.6 | v29.46,4.67 v31.09,6.3 | U4.13 v21.34,5.69 | U6.13 51.82,5.69 49.58,3.45 | v49.17,3.05 49.58,3.45 | v45.72,4.47 40.03,4.47 39.62,4.88 38.81,4.88 38,4.06 38,3.66 37.39,3.05 34.54,3.05 32.72,4.88 v32.72,6.5 | v82.3,5.69 U7.13 | v78.03,5.08 74.57,5.08 v74.37,5.28 74.17,5.28 72.75,3.86 72.75,3.45 73.15,3.05 73.56,3.05 74.17,3.66 74.98,3.66 75.59,3.05 v88.39,3.05 | v60.96,5.69 59.33,4.06 55.88,4.06 55.27,3.45 49.58,3.45 | U8.13 112.78,6.3 v111.15,4.67
SDIN_3V3  (via drill 0.3)
  Top 0.203: v22.15,5.69 22.15,10.16 24.59,12.6 31.09,12.6 33.12,10.57 35.76,10.57 v36.98,11.79 37.8,12.6 v42.47,12.6 | v52.43,5.69 50.8,5.69 45.72,10.77 v45.31,10.77 | v73.36,3.66 60.35,3.66 59.94,4.06 v54.66,4.06 | v112.57,5.28 105.66,5.28 v103.83,3.45
  Bottom 0.203: v36.98,11.79 39.83,11.79 U1.4 | v22.15,5.69 22.15,7.32 U4.14 | v45.31,10.77 43.48,12.6 v42.47,12.6 | U6.14 52.43,7.32 v52.43,5.69 52.43,5.28 53.65,4.06 v54.66,4.06 | 78.84,4.67 78.44,4.67 77.83,4.06 73.76,4.06 v73.36,3.66 | 78.84,4.67 80.47,4.67 80.67,4.47 81.89,4.47 82.91,5.49 82.91,7.32 U7.14 | v112.57,5.28 113.39,6.1 113.39,7.32 U8.14 | v103.83,3.45 90.22,3.45 90.02,3.66 80.67,3.66 80.47,3.45 80.06,3.45 78.84,4.67
SPI_MOSI  (via drill 0.3)
  Top 0.203: v34.34,8.53 33.93,8.53 30.89,11.58 v25.2,11.58
  Bottom 0.203: v34.34,8.53 37.19,8.53 37.59,8.94 37.59,9.35 39.42,11.18 39.83,11.18 U1.5 | v25.2,11.58 24.59,12.19 21.13,12.19 20.12,11.18 17.48,11.18 16.66,10.36 10.57,10.36 9.75,11.18 9.75,12.8 8.53,14.02 SERIAL.8
SPI_SCLK  (via drill 0.3)
  Top 0.203: v33.73,4.88 32.51,3.66 16.46,3.66 8.53,11.58 SERIAL.7
  Bottom 0.203: v33.73,4.88 33.73,6.1 34.54,6.91 38.2,6.91 38.41,7.11 38.41,8.74 39.42,9.75 39.83,9.75 U1.7

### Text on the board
_tsilk: 1 | PCB-DISPARRAY4c | SKAARHOJ 2013 | v10-13

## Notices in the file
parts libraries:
SparkFun: Licensing: CC v3.0 Share-Alike You are welcome to use this library for commercial purposes.
